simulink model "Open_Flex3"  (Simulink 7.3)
settings: Solver=ode4  StartTime=0.0  StopTime=20  RelTol=1e-3
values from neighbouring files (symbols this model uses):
  Ts = 0.04    [run.m]    (also in z2s_transf.m)
undefined symbols (not defined in the file or in its folder): Aol, Bol, Col, Dol

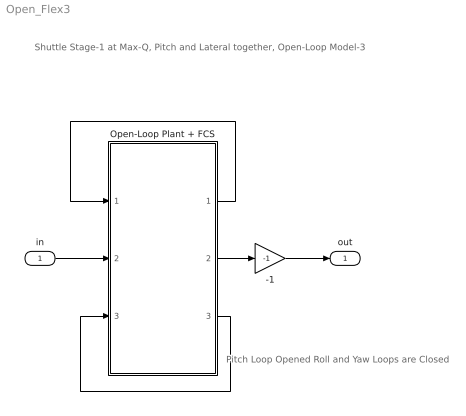
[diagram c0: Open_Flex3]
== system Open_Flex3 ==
  note: Shuttle Stage-1 at Max-Q, Pitch and Lateral together, Open-Loop Model-3
  note: Pitch Loop Opened Roll and Yaw Loops are Closed
  in : Inport  OutDataType=sfix(16)  OutScaling=2^0
  -1 : Gain  Gain=-1  ParameterDataType=sfix(16)  ParameterScaling=2^0  OutDataType=sfix(16)  OutScaling=2^0
  Open-Loop Plant + FCS : Subsystem
  out : Outport  OutDataType=sfix(16)  OutScaling=2^0
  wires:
  -1/1 -> out/1
  Open-Loop Plant + FCS/3(DR_TVC) -> Open-Loop Plant + FCS/3(DR_TVCi)
  in/1 -> Open-Loop Plant + FCS/2(DQ_TVCi)
  Open-Loop Plant + FCS/2(DQ_TVC) -> -1/1
  Open-Loop Plant + FCS/1(DP_TVC) -> Open-Loop Plant + FCS/1(DP_TVCi)

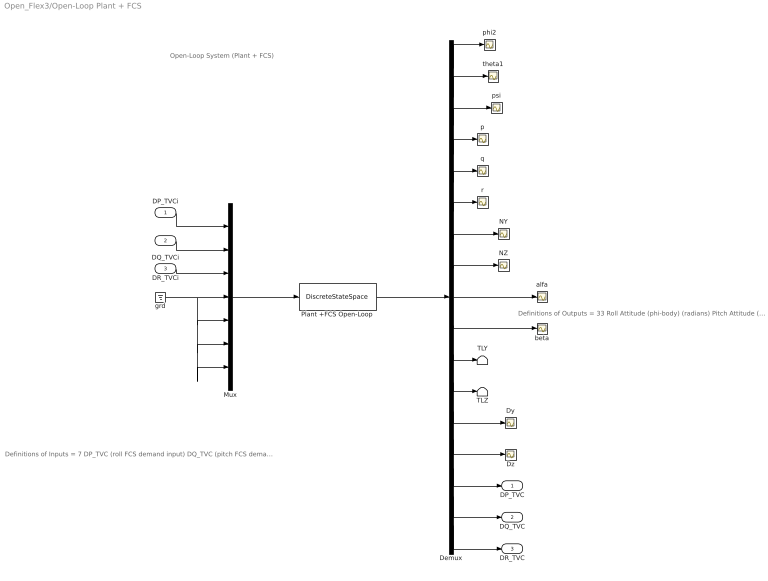
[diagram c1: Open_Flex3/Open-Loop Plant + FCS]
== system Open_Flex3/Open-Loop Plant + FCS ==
  note: Definitions of Outputs = 33 Roll Attitude (phi-body) (radians) Pitch Attitude (thet-bdy) (radians) Yaw Attitude (psi-body) (radians) Roll Rate Gyro (p-flex) (rad/sec) Pitch Rate Gyro (q-flex) (rad/sec) Yaw Rate Gyro (r-flex) (rad/sec) Accelerom # 1, Y-ddot Accelerat. (ft/sec^2) Accelerom # 2, Z-ddot Accelerat. (ft/sec^2) Angle of attack, alfa, (radians) Angle of sideslip, beta, (radian) Load-Torque Pitch TLY-Eng-1 Load-Torque Pitch TLY-Eng-2 Load-Torque Pitch TLY-Eng-3 Load-Torque Pitch TLY-Eng-4 Load-Torque Pitch TLY-Eng-5 Load-Torque Yaw TLZ-Eng-1 Load-Torque Yaw TLZ-Eng-2 Load-Torque Yaw TLZ-Eng-3 Load-Torque Yaw TLZ-Eng-4 Load-Torque Yaw TLZ-Eng-5 Engine # 1 Pitch Deflection dy-1 (rad) Engine # 2 Pitch Deflection dy-2 (rad) Engine # 3 Pitch Deflection dy-3 (rad) Engine # 4 Pitch Deflection dy-4 (rad) Engine # 5 Pitch Deflection dy-5 (rad) Engine # 1 Yaw Deflection dz-1 (rad) Engine # 2 Yaw Deflection dz-2 (rad) Engine # 3 Yaw Deflection dz-3 (rad) Engine # 4 Yaw Deflection dz-4 (rad) Engine # 5 Yaw Deflection dz-5 (rad) DP_TVC (roll FCS demand output) DQ_TVC (pitch FCS demand output) DR_TVC (yaw FCS demand output)
  note: Definitions of Inputs = 7 DP_TVC (roll FCS demand input) DQ_TVC (pitch FCS demand input) DR_TVC (yaw FCS demand input) Wind Gust Velocity (ft/sec) Theta Attitude Command (rad) Phi Attitude Command (rad) Psi Attitude Command (rad)
  note: Open-Loop System (Plant + FCS)
  DP_TVCi : Inport  PortDimensions=1  OutDataType=sfix(16)  OutScaling=2^0
  DQ_TVCi : Inport  Port=2  PortDimensions=1  OutDataType=sfix(16)  OutScaling=2^0
  DR_TVCi : Inport  Port=3  PortDimensions=1  OutDataType=sfix(16)  OutScaling=2^0
  Demux : Demux  Outputs=[1,1,1,1,1,1,1,1,1,1, 5,5,5,5, 1,1,1]
  Dy : Scope
  Dz : Scope
  Mux : Mux  Inputs=7
  NY : Scope
  NZ : Scope
  Plant +FCS Open-Loop : DiscreteStateSpace  A=Aol  B=Bol  C=Col  D=Dol  SampleTime=Ts
  TLY : Terminator
  TLZ : Terminator
  alfa : Scope
  beta : Scope
  grd : Ground
  p : Scope
  phi2 : Scope
  psi : Scope
  q : Scope
  r : Scope
  theta1 : Scope
  DP_TVC : Outport  OutDataType=sfix(16)  OutScaling=2^0
  DQ_TVC : Outport  Port=2  OutDataType=sfix(16)  OutScaling=2^0
  DR_TVC : Outport  Port=3  OutDataType=sfix(16)  OutScaling=2^0
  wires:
  Mux/1 -> Plant +FCS Open-Loop/1
  Demux/7 -> NY/1
  Demux/8 -> NZ/1
  Demux/9 -> alfa/1
  Demux/10 -> beta/1
  Demux/11 -> TLY/1
  Demux/12 -> TLZ/1
  Demux/1 -> phi2/1
  Demux/15 -> DP_TVC/1
  Demux/2 -> theta1/1
  Demux/3 -> psi/1
  Demux/4 -> p/1
  Demux/5 -> q/1
  Demux/6 -> r/1
  Demux/16 -> DQ_TVC/1
  Demux/17 -> DR_TVC/1
  Demux/14 -> Dz/1
  Demux/13 -> Dy/1
  Plant +FCS Open-Loop/1 -> Demux/1
  DP_TVCi/1 -> Mux/1
  DQ_TVCi/1 -> Mux/2
  DR_TVCi/1 -> Mux/3
  grd/1 -> Mux/4, Mux/5, Mux/6, Mux/7
